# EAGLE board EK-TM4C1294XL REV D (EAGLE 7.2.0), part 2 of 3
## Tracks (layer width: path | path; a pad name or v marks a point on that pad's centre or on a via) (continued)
N$31 (continued)
  Top 0.152: 36.27,24.43 Y1.P$3 36.85,24.42 37.11,24.16 38.1,24.16 38.22,24.19 C44.1 | C44.1 38.48,24.17 | C44.1 38.25,24.16 38.18,24.08 38.18,23.47 38.75,22.9 39.44,22.9 39.55,22.78 43.89,22.78 44.42,23.32 44.45,23.32 U1.P$88
N$32
  Top 0.254: U10.P$15 25.7,41.88 26.29,41.3 26.29,40.01 26.14,39.85 23.24,39.85 22.4,40.69 R32.2
N$33
  Top 0.152: 29.26,29.72 30.25,29.72 31.24,30.71 34.82,30.71 35.51,30.02 37.8,30.02 38.1,29.72 38.4,29.72 U1.P$66 | 29.26,29.72 26.29,29.72 26.16,29.59 Y3.P$1 | 29.26,29.72 29.26,29.38 C48.1
N$34
  Top 0.254: U10.P$10 25.91,48.23 26.98,47.17 26.98,39.7 26.67,39.4 22.25,39.4 22.1,39.55 21.64,39.55 R43.2
N$36
  Top 0.254: R45.1 16.3,40.54 | 16.3,40.54 R46.1 | R43.1 20.66,40.53 | 20.66,40.53 20.65,40.54 | 20.66,40.53 20.69,40.5 | 20.69,40.5 R32.1 | 20.69,40.5 20.65,40.77 19.74,40.77 19.51,40.54 19.13,40.54 | 19.13,40.54 16.3,40.54 | C1.1 19.08,40.49 19.13,40.54
N$44
  Top 0.152: U14.4 7.12,45.2 U14.5
  Top 0.254: U14.4 7.07,45.2 6.1,46.18 5.94,46.18 4.65,44.88 4.65,41.99 5.94,40.69 11.73,40.69 12.45,41.4 R45.2
N$45
  Top 0.152: U14.7 7.12,49.28 U14.8
  Top 0.254: U14.8 7.14,49.28 6.1,48.23 6.02,48.23 3.89,46.1 3.89,42.06 5.94,40.01 15.38,40.01 R46.2
PA0  (via drill 0.3)
  Top 0.152: v64.92,26.09 64.95,26.06 67.74,26.06 69.65,24.16 71.93,24.16 72.06,24.18 JP4.2 | v63.27,43.38 62.94,43.05 56.39,43.05 55.85,43.59 50.06,43.59 49.53,43.05 49,43.05 47.49,41.55 U1.P$33 | v63.5,1.75 62.94,2.29 48.08,2.29 47.55,2.82 43.89,2.82 43.59,3.12 42.75,3.12 42.44,2.82 v32.84,2.82 32.99,2.67
  Bottom 0.152: v63.27,43.38 63.25,43.51 63.25,42.06 64.39,40.92 64.39,34.75 63.63,33.98 63.63,33.68 62.79,32.84 62.79,31.85 62.48,31.55 62.48,27.58 64.01,26.06 64.92,26.06 v64.92,26.09 64.92,21.95 63.86,20.8 63.86,6.71 63.55,6.4 63.55,1.83 63.48,1.75 v63.5,1.75 | v32.84,2.82 32.84,2.36 X11.74
PA1  (via drill 0.3)
  Top 0.152: 45.49,44.27 v45.95,44.27 44.35,44.27 44.12,44.04 42.9,44.04 42.29,44.65 38.94,44.65 37.95,43.66 v37.19,43.66 | v69.27,42.22 58.75,42.22 58.22,42.75 55.85,42.75 55.32,43.28 50.22,43.28 49.68,42.75 49.45,42.75 48.54,41.83 48.54,40.92 48.53,40.92 48.23,40.62 47.85,40.62 47.24,41.22 U1.P$34 46.33,42.14 v46.02,42.14
  Bottom 0.152: v46.02,42.14 46.02,42.6 45.95,42.67 v45.95,44.27 | v37.19,43.66 37.19,43.13 36.88,42.82 36.88,40.23 36.12,39.47 36.12,36.96 35.43,36.27 35.43,33.68 34.98,33.22 33.3,33.22 32.16,32.08 32.16,30.56 31.01,29.41 31.01,27.2 29.03,25.22 29.03,14.86 30.02,13.87 30.02,4.8 30.33,4.5 30.33,2.39 X11.76 | JP5.2 71.88,31.75 69.95,33.68 69.95,41.53 v69.27,42.22
PA2  (via drill 0.3)
  Top 0.152: 44,13.56 R20.2 44.04,13.6 44.04,14.02 44.35,14.33 47.47,14.33 47.62,14.48 v49.61,14.48 50.06,14.48 50.29,14.25 52.2,14.25 53.03,13.41 65.68,13.41 66.29,14.02 68.96,14.02 69.65,13.34 v70.56,13.34 | v117.81,6.78 114.38,6.78 114,6.4 113.23,6.4 113.16,6.33 108.89,6.33 108.58,6.02 106.53,6.02 106.22,5.71 97.16,5.71 96.85,6.02 v96.32,6.02 | v96.01,2.59 v71.02,2.59 | U1.P$35 48.31,39.59 v48.31,39.55
  Bottom 0.152: v48.31,39.55 48.31,39.09 48.16,38.94 48.16,34.59 48.92,33.83 48.92,31.47 49.99,30.4 49.99,29.79 49.23,29.03 49.23,25.45 49.91,24.77 49.91,23.55 49.68,23.32 49.68,14.48 v49.61,14.48 | 118.11,1.29 119.18,2.36 119.18,4.42 118.8,4.8 118.8,5.33 117.81,6.33 v117.81,6.78 | v96.32,6.02 96.32,2.9 v96.01,2.59 | v70.56,13.34 70.56,12.88 70.18,12.5 70.18,4.95 71.02,4.12 v71.02,2.59
  Bottom 0.254: 118.11,1.29 X11.6
PA3  (via drill 0.3)
  Top 0.152: v115.14,5.87 115.06,5.79 113.77,5.79 113.69,5.71 109.35,5.71 109.04,5.41 106.98,5.41 106.68,5.11 94.64,5.11 94.49,5.26 93.57,5.26 93.12,4.8 71.86,4.8 71.4,4.34 70.87,4.34 70.18,5.03 69.49,5.03 69.27,4.8 v68.81,4.8 | v68.73,13.26 68.05,13.26 67.82,13.49 66.6,13.49 66.22,13.11 52.88,13.11 52.05,13.95 50.37,13.95 49.61,13.18 v49.23,13.18 48.84,13.56 48.16,13.56 48.12,13.53 48.19,13.38 R19.2 | v46.94,38.63 46.94,39.17 47.32,39.55 47.32,40.01 U1.P$36
  Bottom 0.152: X11.8 115.57,2.31 114.53,3.35 114.53,4.19 115.14,4.8 v115.14,5.87 | v68.81,4.8 68.73,4.88 v68.73,13.26 | v46.94,38.63 46.94,38.1 47.24,37.8 47.24,33.91 48.01,33.15 48.01,28.19 47.4,27.58 47.4,26.36 48.31,25.45 48.31,22.94 49.07,22.17 49.07,16.38 48.31,15.62 48.31,14.1 v49.23,13.18
PA4  (via drill 0.3)
  Top 0.152: v110.11,47.09 109.65,46.63 107.9,46.63 107.59,46.94 90.3,46.94 88.16,44.81 76.96,44.81 75.59,46.18 70.56,46.18 68.66,44.27 62.71,44.27 62.1,43.66 56.84,43.66 56.31,44.2 49.76,44.2 49.23,43.66 46.94,43.66 46.63,43.36 45.41,43.36 | 45.41,43.36 42.06,43.36 41.76,43.66 41.22,43.66 41.17,43.61 v41.22,43.61 | U1.P$37 46.1,40.69 45.41,41.38 45.41,43.36
  Bottom 0.152: v41.22,43.61 41.22,43.66 40.16,44.73 40.16,51.28 X6.18 | X11.10 113.03,2.16 114.22,3.35 114.22,4.12 113.69,4.65 113.69,6.25 114.07,6.63 114.07,35.81 109.73,40.16 109.73,41.83 109.42,42.14 109.42,46.41 109.5,46.48 v110.11,47.09
PA5  (via drill 0.3)
  Top 0.152: v109.04,47.24 90.14,47.24 88.01,45.11 77.19,45.11 75.82,46.48 70.33,46.48 68.43,44.58 62.41,44.58 61.8,43.97 57.15,43.97 56.62,44.5 49.61,44.5 49.07,43.97 46.63,43.97 46.33,43.66 42.52,43.66 41.99,44.2 40.69,44.2 40.46,43.97 | 40.46,43.97 39.7,43.97 v39.29,43.99 | 40.46,43.97 40.46,43.43 40.92,42.98 44.65,42.98 45.11,42.52 45.11,41.07 45.13,41.07 U1.P$38
  Bottom 0.152: X6.20 36.85,52.05 36.85,51.23 39.32,48.77 39.32,44.5 v39.29,43.99 | X11.12 109.5,2.26 109.5,12.95 110.41,13.87 110.41,22.02 109.35,23.09 109.35,24.23 111.1,25.98 111.1,36.35 109.12,38.33 109.12,46.56 109.04,46.63 v109.04,47.24
PA6  (via drill 0.3)
  Top 0.152: X8.16 104.17,50.83 102.41,50.83 101.65,50.06 98.68,50.06 98.37,50.37 v93.88,50.37 93.57,50.06 90.6,50.06 86.87,46.33 78.11,46.33 76.73,47.7 68.73,47.7 67.13,46.1 58.9,46.1 58.37,45.57 55.78,45.57 55.55,45.8 v44.5,45.8 | v44.12,42.37 43.81,42.06 43.81,40.92 44.12,40.62 44.45,40.62 U1.P$40
  Bottom 0.152: v93.88,50.37 92.73,49.23 92.73,25.91 90.98,24.16 90.98,19.58 94.64,15.93 94.64,14.4 93.04,12.8 93.04,5.71 92.73,5.41 92.73,3.83 X11.25 | v44.12,42.37 44.5,42.75 v44.5,45.8
PA7  (via drill 0.3)
  Top 0.152: v90.14,8.15 89.76,8.53 76.89,8.53 76.58,8.23 72.54,8.23 72.24,8.53 v67.59,8.53 66.98,8.53 66.9,8.46 62.56,8.46 62.03,7.85 54.18,7.85 53.14,8.89 X7.8 | v43.2,41 43.97,40.23 44.27,40.23 U1.P$41 | v43.43,45.49 43.74,45.19 44.96,45.19 45.26,45.49 48.84,45.49 49.15,45.19 58.75,45.19 58.98,45.49 v65.46,45.49
  Bottom 0.152: X11.27 90.14,3.83 v90.14,8.15 | v43.2,41 43.2,42.52 43.51,42.82 43.51,44.5 43.43,44.58 v43.43,45.49 | v65.46,45.49 65.46,36.5 68.66,33.3 68.66,28.19 67.97,27.51 67.97,15.24 67.74,15.01 67.74,12.88 67.89,12.72 67.89,12.34 67.74,12.19 67.74,9.14 67.59,8.99 v67.59,8.53
PB0  (via drill 0.3)
  Top 0.152: v54.79,6.02 54.48,5.79 48.31,5.79 48.23,5.71 42.67,5.71 42.6,5.79 v41.3,5.79 41.22,5.87 | R18.1 18.94,22.63 26.36,22.63 30.79,18.21 36.04,18.21 37.26,19.43 41.76,19.43 v42.06,19.74 43.43,21.11 46.18,21.11 47.19,22.12 U1.P$95
  Bottom 0.152: X11.58 52.07,2.16 53.42,3.5 53.42,4.19 54.79,5.56 v54.79,6.02 | v41.3,5.79 39.93,7.16 39.93,7.92 40.46,8.46 40.46,11.51 41.53,12.57 41.53,13.49 41.15,13.87 41.15,16.08 42.06,16.99 v42.06,19.74
PB2  (via drill 0.3)
  Top 0.152: X8.17 102.62,54.61 101.58,53.57 92.2,53.57 v91.44,52.81 | v91.44,51.51 90.22,51.51 85.95,47.24 78.79,47.24 76.5,49.53 67.97,49.53 66.14,47.7 55.24,47.7 54.79,47.32 v47.55,47.32 v38.56,47.32 | v48.31,26.75 48.31,25.07 47.17,23.93 46.79,23.93 46.25,23.39 46.22,23.39 U1.P$91 | v38.71,5.49 v36.2,5.49
  Bottom 0.152: v91.44,52.81 v91.44,51.51 | v47.55,47.32 47.55,44.2 48.46,43.28 48.46,41.15 47.55,40.23 47.55,39.4 47.85,39.09 47.85,34.37 48.62,33.6 48.62,27.81 48.31,27.51 v48.31,26.75 | X11.67 39.37,4.85 v38.71,5.49 | v36.2,5.49 35.2,6.48 35.2,7.7 35.51,8 35.51,10.82 35.81,11.12 35.81,26.82 36.35,27.36 36.35,27.81 35.36,28.8 35.36,31.17 36.2,32 36.2,36.04 36.73,36.58 36.73,39.09 37.49,39.85 37.49,42.14 38.1,42.75 38.1,44.88 37.87,45.11 37.87,46.63 v38.56,47.32
PB3  (via drill 0.3)
  Top 0.152: X8.19 95.45,54.61 94.79,53.95 91.67,53.95 85.57,47.85 79.32,47.85 77.04,50.14 67.36,50.14 65.53,48.31 54.63,48.31 54.56,48.23 47.09,48.23 46.79,48.54 v46.33,48.54 46.02,48.23 43.97,48.23 43.59,48.62 v38.48,48.62 | v49,24 48.54,24 48.16,23.62 47.01,23.62 U1.P$92
  Bottom 0.152: v46.33,48.54 46.33,44.88 48.08,43.13 48.08,41.38 47.24,40.54 47.24,39.24 47.55,38.94 47.55,34.14 48.31,33.38 48.31,28.04 47.7,27.43 47.7,26.52 48.62,25.6 48.62,25.07 49,24.69 v49,24 | X11.69 36.83,3.86 35.36,5.33 35.05,5.33 34.44,5.94 34.44,7.47 35.13,8.15 35.13,11.2 35.43,11.51 35.43,26.21 34.9,26.75 34.9,31.39 35.81,32.31 35.81,36.2 36.42,36.8 36.42,39.24 37.19,40.01 37.19,42.44 37.8,43.05 37.8,44.65 37.57,44.88 37.57,47.7 v38.48,48.62
PB4  (via drill 0.3)
  Top 0.152: v94.03,12.65 v78.56,12.65 | v94.03,4.65 94.56,4.65 94.72,4.8 106.91,4.8 107.21,5.11 109.19,5.11 109.5,5.41 113.92,5.41 114,5.49 114.68,5.49 114.91,5.26 117.65,5.26 v117.81,5.41 | v78.56,26.75 76.5,26.75 75.29,27.96 71.25,27.96 70.56,27.28 57.84,27.28 57.07,28.04 57.03,28.04 U1.P$121 55.85,29.21 55.85,29.87 56.24,30.25 v56.24,30.94
  Bottom 0.152: v78.56,12.65 78.56,17.6 78.87,17.91 78.87,20.04 78.56,20.34 v78.56,26.75 | v94.03,12.65 v94.03,4.65 | v117.81,5.41 117.81,4.95 118.11,4.65 X11.5 | X6.6 54.61,50.88 53.87,50.14 53.87,44.27 54.41,43.74 54.41,33.07 56.24,31.24 v56.24,30.94
PB5  (via drill 0.3)
  Top 0.152: v116.05,5.87 116.05,6.48 114.83,6.48 114.45,6.1 113.46,6.1 113.39,6.02 109.12,6.02 108.81,5.71 106.76,5.71 106.45,5.41 94.87,5.41 94.72,5.56 93.34,5.56 93.19,5.41 86.87,5.41 86.56,5.11 71.25,5.11 v71.09,5.03 | v69.57,26.67 68.5,26.67 68.2,26.98 57.68,26.98 56.92,27.74 56.77,27.74 U1.P$120 55.47,29.03 55.47,30.1 v54.71,30.86
  Bottom 0.152: X11.7 115.57,5.38 v116.05,5.87 | v71.09,5.03 71.09,8.38 71.48,8.76 71.48,20.88 70.56,21.79 70.56,23.62 71.09,24.16 71.09,25.15 v69.57,26.67 | X6.8 52.07,51.03 52.88,50.22 52.88,43.74 53.49,43.13 53.49,32.16 v54.71,30.86
PC4  (via drill 0.3)  (1 unrouted)
  Top 0.152: v98.22,48.54 100.51,48.54 100.81,48.84 101.88,48.84 102.18,48.54 109.88,48.54 111.18,49.84 v117.96,49.84 | v95.33,37.57 94.87,37.57 94.72,37.72 85.04,37.72 84.2,36.88 78.33,36.88 77.5,37.72 71.09,37.72 67.51,41.3 57.99,41.3 57.91,41.38 52.73,41.38 52.27,40.92 52.27,40.2 U1.P$25
  Bottom 0.152: v98.22,48.54 98.3,40.84 98.3,39.55 96.32,37.57 v95.33,37.57 95.33,31.24 96.62,29.95 96.62,28.42 96.39,28.19 96.39,26.98 96.55,26.82 99.44,23.85 99.44,19.13 95.33,15.01 95.33,3.89 X11.23 | v117.96,49.84 117.96,50.37 119.18,51.59 119.18,53.54 X8.5
PC5  (via drill 0.3)  (1 unrouted)
  Top 0.152: v99.06,47.93 100.43,47.93 101.04,48.54 101.65,48.54 101.96,48.23 110.41,48.23 110.72,48.54 111.33,49.23 v116.74,49.23 | v97.54,37.26 97.08,37.26 96.77,36.96 95.02,36.96 94.56,37.41 85.27,37.41 84.43,36.58 78.11,36.58 77.27,37.41 70.87,37.41 67.28,41 57.76,41 57.68,41.07 52.88,41.07 52.58,40.77 52.58,39.94 U1.P$24
  Bottom 0.152: X8.7 115.57,53.67 116.74,52.5 v116.74,49.23 | v99.06,47.93 99.06,39.01 97.54,37.49 v97.54,37.26 97.54,28.5 100.36,25.68 100.36,18.67 99.9,18.21 99.9,15.54 99.59,15.24 99.59,13.34 98.53,12.27 98.53,5.79 97.54,4.8 97.54,4.04 97.74,3.83 97.77,3.83 X11.21
PC6  (via drill 0.3)  (1 unrouted)
  Top 0.152: v111.48,48.16 111.25,47.93 v101.35,47.93 | v100.81,37.03 100.43,36.65 94.79,36.65 94.34,37.11 85.5,37.11 84.66,36.27 77.8,36.27 76.96,37.11 70.64,37.11 67.06,40.69 57.61,40.69 57.53,40.77 53.11,40.77 52.88,40.54 52.88,39.67 U1.P$23
  Bottom 0.152: X8.9 112.01,53.59 112.01,48.69 v111.48,48.16 | v101.35,47.93 101.35,40.62 101.19,40.46 101.19,37.41 v100.81,37.03 100.81,34.82 100.58,34.52 100.58,27.43 103.1,24.92 103.1,14.33 101.35,12.57 101.35,4.95 100.33,3.94 X11.19
PC7  (via drill 0.3)  (1 unrouted)
  Top 0.152: v101.8,37.49 101.8,36.96 101.19,36.35 94.56,36.35 94.11,36.8 85.72,36.8 84.89,35.97 77.57,35.97 76.73,36.8 70.41,36.8 66.83,40.39 57.45,40.39 57.38,40.46 53.34,40.46 53.19,40.31 53.19,39.41 U1.P$22
  Bottom 0.152: X11.17 102.87,7.09 101.8,8.15 101.8,12.5 103.4,14.1 103.4,25.22 100.97,27.66 100.97,32.38 101.8,33.22 v101.8,37.49 101.5,37.8 101.5,40.08 101.8,40.39 101.8,47.32 101.96,47.47 101.96,49.61 104.09,51.74 104.09,53.29 X8.15
PD0  (via drill 0.3)
  Top 0.152: X9.14 107.95,8.74 107.06,7.85 104.93,7.85 104.62,7.54 99.67,7.54 98.91,8.31 92.73,8.31 91.67,7.24 86.33,7.24 85.72,7.85 84.35,7.85 84.12,7.62 78.41,7.62 77.72,6.93 70.18,6.93 69.49,7.62 66.45,7.62 66.22,7.85 63.86,7.85 v63.25,7.24 | v62.18,32.23 61.87,32.54 58.65,32.54 U1.P$1
  Bottom 0.152: X11.50 63.25,2.36 v63.25,7.24 63.25,8.53 63.55,8.84 63.55,21.03 64.62,22.17 64.62,24.92 62.18,27.36 v62.18,32.23
PD1  (via drill 0.3)
  Top 0.152: X9.12 110.49,8 110.34,7.85 107.67,7.85 107.37,7.54 105.31,7.54 105,7.24 99.52,7.24 98.75,8 92.96,8 91.9,6.93 86.03,6.93 85.42,7.54 84.66,7.54 84.35,7.24 78.56,7.24 77.95,6.63 69.95,6.63 69.34,7.24 v65.84,7.24 | v65.99,33.53 63.78,33.53 63.09,32.84 59.74,32.84 58.9,33.68 58.77,33.68 U1.P$2
  Bottom 0.152: X11.48 64.8,1.29 64.85,1.29 65.84,2.29 v65.84,7.24 65.84,8.46 65.99,8.61 v65.99,33.53
PD2  (via drill 0.3)
  Top 0.152: v60.73,33.45 59.59,33.45 59.05,33.98 58.51,33.98 U1.P$3
  Bottom 0.152: X6.3 58.67,53.09 58.67,51.13 60.5,49.3 v60.73,33.45 60.73,32.46 61.87,31.39 61.87,27.13 64.31,24.69 64.31,22.33 63.25,21.18 61.87,19.81 61.87,4.95 61.19,4.27 61.19,2.77 X11.52
PD3  (via drill 0.3)
  Top 0.152: X8.13 107.95,54.46 106.68,53.19 93.04,53.19 v92.81,52.96 | v92.81,51.44 92.28,50.9 90.22,50.9 86.26,46.94 78.56,46.94 76.5,49 72.39,49 71.7,48.31 68.35,48.31 66.83,46.79 57.76,46.79 57.45,46.48 v56.31,46.48 | 56.16,32.99 v56.27,32.99 56.92,32.99 57.15,33.22 57.18,33.22 U1.P$4 | v57.99,19.89 59.21,19.89 59.66,20.19 v66.75,20.19
  Bottom 0.152: v92.81,52.96 v92.81,51.44 | v66.75,20.19 66.75,13.41 66.52,13.18 66.52,4.65 66.22,4.34 66.22,2.36 X11.46 | v57.99,19.89 57.99,20.5 57.91,20.57 57.91,26.75 56.92,27.74 56.92,31.17 56.24,31.85 56.24,32.92 v56.27,32.99 56.31,33.1 v56.31,46.48
PD4  (via drill 0.3)  (1 unrouted)
  Top 0.152: v73.15,29.18 70.71,29.18 70.03,28.5 60.88,28.5 60.27,29.11 58.22,29.11 U1.P$125
  Bottom 0.152: X11.40 73.84,2.36 73.84,25.58 JP4.3 73.15,28.45 v73.15,29.18
PD5  (via drill 0.3)  (1 unrouted)
  Top 0.152: v74.37,29.18 74.37,29.26 73.84,29.79 70.71,29.79 69.72,28.8 61.11,28.8 60.5,29.41 58.52,29.41 58.37,29.57 58.33,29.57 U1.P$126
  Bottom 0.152: X11.38 76.43,2.31 76.43,5.64 75.59,6.48 75.59,20.19 76.2,20.8 76.2,27.36 v74.37,29.18 73.84,29.72 73.84,33.22 74.91,34.29 JP5.3
PD6  (via drill 0.3)
  Top 0.152: U4.4 77.57,41.45 v77.57,40.54 | v76.96,29.72 74.98,29.72 74.6,30.1 70.03,30.1 v69.34,29.41 69.34,29.49 68.89,29.49 68.5,29.11 61.34,29.11 60.73,29.72 58.75,29.72 58.6,29.87 58.59,29.87 U1.P$127
  Bottom 0.152: v77.57,40.54 77.57,39.85 77.5,39.78 77.5,31.24 76.96,30.71 v76.96,29.72 | v69.34,29.41 69.34,28.35 68.28,27.28 68.28,15.01 68.12,14.86 68.12,13.03 68.43,12.72 68.43,11.73 68.12,11.43 68.12,9.22 68.35,8.99 68.35,8.08 68.12,7.85 68.12,4.5 68.81,3.81 68.81,2.31 X11.44
PD7  (via drill 0.3)
  Top 0.152: X8.14 107.09,52.07 105.54,50.52 102.79,50.52 102.03,49.76 90.91,49.76 87.17,46.02 77.8,46.02 76.43,47.4 68.89,47.4 66.37,44.88 v59.36,44.88 | v60.5,30.86 58.67,30.86 U1.P$128 | X11.42 71.42,1.27 69.95,2.74 58.67,2.74 v58.45,2.97
  Bottom 0.152: v59.36,44.88 59.36,43.81 59.13,43.59 59.13,35.97 59.28,35.81 59.28,32 60.43,30.86 v60.5,30.86 59.82,30.18 59.82,25.38 60.58,24.61 60.58,22.55 61.19,21.95 61.19,7.16 58.45,4.42 v58.45,2.97
PE0  (via drill 0.3)
  Top 0.152: X11.14 109.04,1.27 109.35,1.6 109.96,2.29 117.04,2.29 v117.12,2.21 | v66.06,37.34 65.23,38.18 59.97,38.18 59.21,37.41 55.17,37.41 54.71,36.96 54.69,36.96 U1.P$15 | X8.6 116.18,50.14 110.95,50.14 109.65,48.84 102.49,48.84 102.18,49.15 91.44,49.15 87.71,45.41 77.42,45.41 76.05,46.79 70.1,46.79 68.73,45.41 v68.2,45.41
  Bottom 0.152: X8.6 118.11,51.05 117.27,50.22 117.27,49.61 117.35,49.53 117.35,46.41 116.81,45.87 116.81,44.5 117.04,44.27 117.04,38.25 115.9,37.11 115.9,33.22 118.42,30.71 118.42,25.6 117.65,24.84 117.65,12.57 117.12,12.04 v117.12,2.21 | v66.06,37.34 66.45,37.34 67.28,38.18 67.28,44.5 v68.2,45.41
PE1  (via drill 0.3)
  Top 0.152: X11.16 106.45,1.27 106.91,1.75 107.44,2.29 109.5,2.29 109.8,2.59 116.2,2.59 v116.51,2.9 | v66.67,36.2 66.29,36.2 64.62,37.87 60.12,37.87 59.36,37.11 55.41,37.11 U1.P$14 | X8.8 114.17,50.67 106.83,50.67 105.31,49.15 102.87,49.15 102.56,49.45 91.14,49.45 87.4,45.72 77.65,45.72 76.28,47.09 69.88,47.09 69.49,46.71 v69.04,46.71
  Bottom 0.152: X8.8 116.05,51.59 116.05,48.23 116.43,47.85 116.51,47.78 116.51,44.35 116.74,44.12 116.74,38.48 115.21,36.96 115.21,33.3 118.11,30.4 118.11,25.83 117.35,25.07 117.35,12.8 116.66,12.12 116.66,3.05 v116.51,2.9 | v66.67,36.2 67.67,37.19 67.67,43.43 69.04,44.81 v69.04,46.71
PE2  (via drill 0.3)
  Top 0.152: v103.94,37.72 103.25,37.03 102.49,37.03 101.42,35.97 89.92,35.97 88.7,34.75 76.5,34.75 75.67,35.59 66.29,35.59 64.31,37.57 60.35,37.57 59.59,36.8 55.7,36.8 55.32,36.42 55.24,36.42 55.03,36.2 U1.P$13 | X8.10 112.88,52.07 111.78,50.98 106.53,50.98 105.69,50.14 103.4,50.14 v103.1,49.84
  Bottom 0.152: v103.1,49.84 102.26,49 102.26,42.06 104.24,40.08 104.24,38.02 v103.94,37.72 103.94,2.44 102.87,1.37 X11.18
PE3  (via drill 0.3)
  Top 0.152: v109.8,19.51 109.65,19.36 104.78,19.36 103.56,18.14 v102.18,18.14 | U1.P$12 55.93,36.5 59.74,36.5 60.5,37.26 64.08,37.26 66.06,35.28 75.44,35.28 76.28,34.44 88.92,34.44 90.14,35.66 101.65,35.66 102.64,36.65 103.94,36.65 104.7,37.41 104.7,39.93 106.6,41.83 v108.43,41.83
  Bottom 0.152: X8.12 110.49,50.44 108.36,48.31 108.36,42.75 108.43,42.67 v108.43,41.83 108.43,39.4 108.66,39.17 108.66,38.18 110.8,36.04 110.8,26.36 108.97,24.54 108.97,22.78 109.8,21.95 v109.8,19.51 | v102.18,18.14 101.42,17.37 101.42,14.1 99.21,11.89 99.21,2.39 X11.20
PE4  (via drill 0.3)
  Top 0.152: v100.81,17.53 115.21,17.53 116.59,16.15 v119.33,16.15 | 79.4,27.43 v79.32,27.43 76.43,27.43 75.59,28.27 70.94,28.27 70.56,27.89 60.5,27.89 59.89,28.5 57.7,28.5 U1.P$123 | v101.35,24.61 100.13,25.83 98.98,25.83 98.68,26.14 92.51,26.14 89.46,23.09 v79.4,23.09
  Bottom 0.152: X8.3 120.52,54.61 119.56,53.65 119.56,51.44 118.57,50.44 118.57,45.95 118.34,45.72 118.34,38.79 120.17,36.96 120.17,31.62 118.72,30.18 118.72,16.76 v119.33,16.15 | X11.22 98.83,2.31 98.83,12.04 100.81,14.02 v100.81,17.53 101.35,18.06 101.35,18.21 102.49,19.36 102.49,23.47 v101.35,24.61 | v79.4,23.09 79.4,27.36 v79.32,27.43
PE5  (via drill 0.3)
  Top 0.152: v108.05,29.34 108.05,28.88 105.99,26.82 101.8,26.82 100.66,27.96 99.14,27.96 98.6,27.43 v97.08,27.43 91.21,27.43 90.68,27.96 79.7,27.96 79.63,28.04 79.02,28.04 78.94,27.96 76.43,27.96 75.82,28.57 70.64,28.57 70.26,28.19 60.66,28.19 60.05,28.8 57.99,28.8 57.76,29.03 57.73,29.03 U1.P$124
  Bottom 0.152: X8.11 109.5,53.62 109.5,50.06 108.05,48.62 108.05,42.6 107.52,42.06 107.52,41.6 108.05,41.07 108.05,38.79 108.36,38.48 108.36,35.74 109.65,34.44 109.65,30.86 108.13,29.34 v108.05,29.34 | v97.08,27.43 97.08,26.9 99.75,24.23 99.75,18.97 99.29,18.52 99.29,18.36 97.23,16.31 97.23,4.72 96.77,4.19 96.77,1.83 96.24,1.29 95.63,1.29 95.56,1.22 X11.24
PF0  (via drill 0.3)
  Top 0.152: D4.A 32.91,6.24 v33.3,6.63 33.38,6.71 39.4,6.71 v40.39,5.71 | v39.09,13.79 34.82,13.79 34.67,13.79 v33.3,13.79 | v41.38,41.91 41.99,41.3 41.99,41 42.22,40.77 43.05,39.85 44.09,39.85 U1.P$42
  Bottom 0.152: v39.09,13.79 39.09,14.63 38.86,14.86 38.86,18.9 40.01,20.12 40.92,21.03 40.92,22.86 40.01,23.77 40.01,33.68 41.07,34.75 41.07,36.73 40.54,37.26 40.54,40.23 41.38,41.07 v41.38,41.91 | v33.3,13.79 33.3,10.29 33.38,10.21 33.38,7.32 33.3,7.24 v33.3,6.63 | X11.66 41.91,1.91 40.62,3.2 40.62,5.49 v40.39,5.71
PF1  (via drill 0.3)
  Top 0.152: X9.1 123.19,13.44 121.08,15.54 116.51,15.54 114.83,17.22 101.88,17.22 101.58,16.92 98.6,16.92 97.99,16.31 93.12,16.31 92.89,16.08 v92.05,16.08 | v90.53,31.55 89.92,31.55 89.53,31.17 81.46,31.17 81,30.71 69.04,30.71 68.12,29.79 63.48,29.79 61.49,31.77 56.69,31.77 56.39,32.08 54.86,32.08 54.33,32.61 52.43,32.61 52.12,32.92 46.79,32.92 v46.25,32.38 | v46.18,38.18 45.72,38.18 45.57,38.02 45.34,38.02 45.26,38.1 45.26,38.11 U1.P$43 | v47.85,18.97 47.55,18.67 44.04,18.67 43.28,17.91 38.86,17.91 v38.25,17.3
  Bottom 0.152: v92.05,16.08 90.37,17.75 90.37,24.46 91.29,25.38 91.29,26.67 91.06,26.9 91.06,30.18 90.53,30.71 v90.53,31.55 | v46.18,38.18 46.18,37.64 45.95,37.41 45.95,36.73 46.63,36.04 46.63,32.77 v46.25,32.38 46.79,31.85 46.79,31.39 46.33,30.94 46.33,26.06 47.4,24.99 47.4,22.4 48.16,21.64 48.16,19.81 47.85,19.51 v47.85,18.97 | v38.25,17.3 38.25,12.88 38.33,12.8 38.33,6.86 38.1,6.63 38.1,5.03 38.33,4.8 38.33,3.35 38.63,3.05 38.63,1.98 39.34,1.27 X11.68
PF2  (via drill 0.3)
  Top 0.152: 120.62,11.4 120.62,12.27 119.41,13.49 117.88,13.49 114.45,16.92 102.11,16.92 101.5,16.31 v98.98,16.31 | v96.77,30.79 88.09,30.79 88.01,30.86 81.69,30.86 81.23,30.4 69.27,30.4 68.35,29.49 63.25,29.49 61.27,31.47 56.54,31.47 56.24,31.77 54.56,31.77 54.03,32.31 52.2,32.31 51.89,32.61 47.7,32.61 v47.4,32.31 | v46.56,37.11 46.1,37.57 45.24,37.57 U1.P$44 | v44.58,6.33 43.28,6.33 43.2,6.4 40.31,6.4 39.4,7.32 v37.72,7.32 | 120.62,11.35 120.62,11.4 | 120.62,11.4 X9.3
  Bottom 0.152: v98.98,16.31 98.98,17.37 99.59,17.98 99.59,18.36 100.05,18.82 100.05,25.45 96.93,28.57 96.93,30.63 v96.77,30.79 | v46.56,37.11 46.94,36.73 46.94,32.77 v47.4,32.31 47.4,31.47 46.63,30.71 46.63,26.21 47.7,25.15 47.7,22.63 48.46,21.87 48.46,16.69 46.02,14.25 46.02,11.96 45.87,11.81 45.87,10.97 46.33,10.52 46.33,9.68 45.87,9.22 45.87,7.62 v44.58,6.33 | v37.72,7.32 37.72,4.65 38.02,4.34 38.02,1.68 37.8,1.45 37.34,1.45 37.29,1.4 37.11,1.4 X11.70
PF3  (via drill 0.3)
  Top 0.152: X9.5 113.84,15.7 v93.88,15.7 | v90.22,45.87 89.76,45.34 89.23,45.34 88.39,44.5 76.81,44.5 75.44,45.87 70.79,45.87 68.89,43.97 62.94,43.97 62.33,43.36 56.54,43.36 56.01,43.89 49.91,43.89 49.38,43.36 47.62,43.36 v47.09,42.82 | v45.19,36.96 45.19,37.03 44.1,38.12 U1.P$45 | v34.75,32.23 36.42,32.23 37.11,31.55 39.47,31.55 39.55,31.47 44.42,31.47 44.73,31.77 45.34,31.77 45.41,31.85 v45.49,31.85
  Bottom 0.152: v90.22,45.87 90.22,39.09 92.2,37.11 92.2,31.39 91.36,30.56 91.36,27.81 91.59,27.58 91.59,25.22 90.68,24.31 90.68,18.9 v93.88,15.7 | v47.09,42.82 46.71,42.44 46.71,40.69 45.19,39.17 v45.19,36.96 46.25,35.89 46.25,33.3 45.49,32.54 v45.49,31.85 45.41,31.85 | X11.72 34.29,2.29 35.28,3.28 35.28,4.57 34.06,5.79 34.06,19.43 34.52,19.89 34.52,31.55 34.75,31.77 v34.75,32.23
PF4  (via drill 0.3)
  Top 0.152: X11.64 44.45,1.4 44.27,1.37 44.2,1.45 43.28,1.45 42.44,2.29 38.79,2.29 38.56,2.06 37.64,2.06 37.41,2.29 33.38,2.29 33.22,2.13 32.54,2.13 32.38,2.29 28.35,2.29 v27.96,1.91 | v27.96,6.1 29.07,6.1 D3.A | v45.03,36.04 45.03,36.2 44.58,36.65 44.58,37.11 U1.P$46 | v44.73,32.38 44.2,32.38 44.04,32.23 43.36,32.23 42.9,31.77 39.78,31.77 39.7,31.85 37.41,31.85 36.35,32.92 34.59,32.92 34.14,32.46 34.14,32.31 33.76,31.93 31.85,31.93 v30.86,32.92
  Bottom 0.152: v27.96,1.91 v27.96,6.1 27.96,6.63 27.81,6.78 27.81,12.65 27.05,13.41 27.05,26.36 28.04,27.36 29.57,28.88 29.57,29.79 30.86,31.09 v30.86,32.92 | v45.03,36.04 45.87,35.2 45.87,33.45 44.81,32.38 v44.73,32.38
PG0  (via drill 0.3)
  Top 0.152: 115.59,11.43 111.63,15.39 98.15,15.39 97.84,15.09 93.34,15.09 92.96,15.47 90.3,15.47 87.86,17.91 86.64,17.91 v86.33,18.21 86.18,18.21 85.88,17.91 80.54,17.91 79.78,18.67 79.02,18.67 77.95,17.6 76.5,17.6 76.2,17.91 73.69,17.91 73.3,18.29 70.18,18.29 69.88,18.59 69.04,18.59 68.81,18.36 52.5,18.36 51.89,18.97 49.23,18.97 48.31,19.89 46.86,19.89 v46.63,19.58 | 43.81,36.16 v44.12,36.04 | v44.12,36.04 43.97,36.04 44.08,36.09 v44.12,36.04 | U1.P$49 43.94,36.04 v44.12,36.04
  Top 0.254: 115.59,11.43 X9.7
  Bottom 0.152: v86.33,18.21 86.33,17.53 86.11,17.3 86.11,13.49 85.42,12.8 85.42,7.47 85.65,7.24 85.65,6.55 85.11,6.02 85.11,3.83 X11.31 | v46.63,19.58 46.63,22.55 45.72,23.47 45.72,25.76 45.64,25.83 45.64,28.04 45.11,28.57 45.11,31.17 44.12,32.16 44.12,32.69 44.58,33.15 45.03,33.15 45.41,33.53 45.41,35.2 45.26,35.36 44.81,35.36 v44.12,36.04
PG1  (via drill 0.3)
  Top 0.152: v87.63,12.04 87.55,11.96 62.87,11.96 62.71,12.12 60.38,12.12 X7.1 | v57,32.38 55.09,32.38 53.65,33.83 51.82,33.83 50.29,35.43 43.66,35.43 43.28,35.81 43.28,36.12 42.69,36.71 U1.P$50 | v59.82,16.54 59.51,16.84 58.06,16.84 v57.76,16.54
  Bottom 0.152: X11.29 v87.63,12.04 | v57,32.38 57,31.62 57.23,31.39 57.23,27.89 58.22,26.9 58.22,20.95 58.6,20.57 58.6,18.36 57.76,17.53 57.76,16.56 57.73,16.56 v57.76,16.54 | X7.1 60.27,12.01 60.27,16.08 v59.82,16.54
PH0  (via drill 0.3)
  Top 0.152: v113.16,7.01 112.78,6.63 108.66,6.63 108.36,6.33 106.3,6.33 105.99,6.02 98.91,6.02 98.15,6.78 94.03,6.78 92.96,5.71 82.07,5.71 81.15,6.63 78.87,6.63 78.26,6.02 63.02,6.02 62.1,6.93 54.1,6.93 53.57,6.4 49.23,6.4 48.39,7.24 46.02,7.24 45.72,7.54 43.66,7.54 43.59,7.62 v43.13,7.62 | 50.44,40.69 50.44,40.62 | v49.15,38.33 49.15,39.55 49.53,39.93 49.76,39.93 50.44,40.61 50.44,40.62 | v48.84,34.82 48.54,35.13 45.72,35.13 45.34,34.75 v44.81,34.75 | U1.P$29 50.44,40.62
  Bottom 0.152: 112.93,3.81 X11.9 | 113.08,3.81 113.16,3.89 v113.16,7.01 | v43.13,7.62 43.43,7.92 43.43,10.41 X7.13 44.42,11.58 44.42,11.43 43.66,12.19 43.66,15.09 45.03,16.46 45.03,22.02 44.42,22.63 44.42,24.84 43.66,25.6 43.66,27.81 44.5,28.65 44.5,30.86 43.51,31.85 43.51,32.99 44.2,33.68 44.2,34.21 44.73,34.75 v44.81,34.75 | v49.15,38.33 49.15,37.87 48.46,37.19 48.46,35.2 v48.84,34.82 48.92,34.82
  Bottom 0.254: 113.08,3.81 X11.9
PH1  (via drill 0.3)
  Top 0.152: v112.24,7.24 111.94,6.93 108.43,6.93 108.13,6.63 106.07,6.63 105.77,6.33 99.06,6.33 98.3,7.09 93.8,7.09 92.73,6.02 82.3,6.02 81.38,6.93 78.72,6.93 78.11,6.33 63.25,6.33 62.33,7.24 53.87,7.24 53.34,6.71 49.38,6.71 48.54,7.54 46.25,7.54 45.95,7.85 43.97,7.85 43.51,8.31 42.9,8.31 42.37,7.77 v40.92,7.77 | v42.44,45.57 43.13,44.88 45.11,44.88 45.41,45.19 46.48,45.19 46.79,44.88 v48.31,44.88 | v48.92,40.39 49.63,40.39 U1.P$30
  Bottom 0.152: X11.11 110.57,3.81 110.49,4.42 X11.11 | X11.11 111.48,4.8 111.48,6.48 v112.24,7.24 | v40.92,7.77 40.92,10.44 X7.15 42.67,12.19 42.98,12.19 42.98,15.47 43.89,16.38 43.89,19.96 43.81,20.04 43.81,20.65 44.12,20.95 44.12,24.54 43.36,25.3 43.36,27.96 44.2,28.8 44.2,30.71 43.2,31.7 43.2,33.15 43.89,33.83 43.89,35.36 43.43,35.81 43.43,36.58 44.58,37.72 44.58,38.79 42.6,40.77 42.6,42.44 43.2,43.05 43.2,44.2 42.44,45.03 v42.44,45.57 | v48.31,44.88 48.31,44.35 48.84,43.81 48.84,40.39 v48.92,40.39
PH2  (via drill 0.3)
  Top 0.152: v118.64,6.4 118.64,5.11 118.34,4.8 115.14,4.8 114.61,4.27 114.07,4.27 113.54,4.8 109.96,4.8 109.04,3.89 108.03,3.89 X11.13 | v102.41,16.31 114.38,16.31 117.81,12.88 v119.02,12.88 | v98.98,37.57 98.37,38.18 94.94,38.18 94.79,38.02 84.81,38.02 83.97,37.19 78.56,37.19 77.72,38.02 71.32,38.02 67.74,41.6 58.14,41.6 57.61,42.14 55.24,42.14 54.71,42.67 50.67,42.67 50.52,42.52 50.52,41.83 U1.P$31
  Bottom 0.152: v118.64,6.4 118.64,8.36 X9.6 119.18,9.96 119.18,12.12 119.02,12.27 v119.02,12.88 | 98.98,37.49 v98.98,37.57 98.98,36.73 98.68,36.42 98.68,33.76 100.28,32.16 100.28,27.13 102.79,24.61 102.79,17.75 102.41,17.37 v102.41,16.31
PH3  (via drill 0.3)
  Top 0.152: 105.41,3.83 X11.15 106.45,3.81 107.44,4.8 109.5,4.8 109.8,5.11 114.15,5.11 v114.38,4.88 | U1.P$32 49.45,41.73 49.45,41.99 50.44,42.98 55.02,42.98 55.55,42.44 57.91,42.44 58.45,41.91 67.97,41.91 71.55,38.33 77.95,38.33 78.79,37.49 83.74,37.49 84.58,38.33 94.49,38.33 94.64,38.48 98.22,38.48 102.18,42.44 v110.03,42.44
  Bottom 0.152: X9.8 114.99,8.31 114.99,6.63 114.38,6.02 v114.38,4.88 | 115.59,8.91 X9.8 | X11.15 105.39,3.81 105.31,3.89 | X9.8 114.53,9.93 114.53,35.81 110.03,40.31 v110.03,42.44
PJ0  (via drill 0.3)
  Top 0.152: USR_SW1.P$2 6.33,7.62 6.55,7.39 v7.62,7.39 8.91,6.1 15.32,6.1 v19.36,10.13 19.81,10.13 20.88,11.2 23.39,11.2 27.96,15.77 41.07,15.77 41.68,16.38 44.42,16.38 45.19,17.14 50.67,17.14 51.36,16.46 54.41,16.46 v54.71,16.15 | v52.65,30.4 52.73,29.26 53.72,28.27 53.95,28.27 55.01,27.21 U1.P$116 | USR_SW1.P$1 6.38,15.32 6.71,15.32 6.71,15.47 v8.38,15.47
  Bottom 0.152: X11.82 20.57,2.29 20.57,5.56 19.36,6.78 v19.36,10.13 | v52.65,30.4 52.73,30.33 52.73,29.72 54.06,28.38 54.06,24.73 54.03,24.69 54.03,23.32 55.02,22.33 55.02,16.99 54.71,16.69 v54.71,16.15 | v8.38,15.47 8.38,14.25 7.62,13.49 v7.62,7.39
PJ1  (via drill 0.3)  (1 unrouted)
  Top 0.152: v55.93,16.46 55.55,16.76 51.51,16.76 50.83,17.45 44.96,17.45 44.2,16.69 41.45,16.69 40.84,16.08 27.74,16.08 23.16,11.51 19.2,11.51 18.52,10.82 v14.25,10.82 14.25,8.59 USR_SW2.P$2 | v14.25,12.65 14.25,13.95 14.55,14.51 USR_SW2.P$1 | v54.03,30.25 54.03,29.79 54.1,29.72 54.1,28.7 U1.P$117
  Bottom 0.152: X11.84 17.98,2.34 v17.98,10.82 | v14.25,10.82 v14.25,12.65 | v55.93,16.46 56.24,16.76 56.24,18.75 55.63,19.36 55.63,22.63 57,24 57,25.53 55.55,26.9 55.55,29.03 55.47,29.11 54.63,29.11 54.25,29.49 54.25,30.18 54.18,30.25 v54.03,30.25
PK0  (via drill 0.3)
  Top 0.152: v68.28,36.27 68.28,36.35 68.12,36.5 68.12,36.58 65.53,39.17 56.84,39.17 56.77,39.24 54.56,39.24 54.41,39.09 54.41,38.37 U1.P$18 53.58,37.57 52.27,36.27 v52.27,35.97 | v70.79,10.52 v92.05,10.52
  Bottom 0.152: X11.26 91.67,2.31 91.67,10.13 v92.05,10.52 | v52.27,35.97 52.27,36.42 53.19,37.34 53.19,42.9 52.58,43.51 52.5,49.99 50.49,51.99 49.61,51.99 X6.10 | 68.58,35.97 v68.28,36.27 69.27,35.28 69.27,32.92 70.03,32.16 70.03,28.57 68.58,27.13 68.58,23.24 69.72,23.24 70.26,22.71 70.26,21.57 71.17,20.65 71.17,11.43 70.79,11.05 v70.79,10.52
PK1  (via drill 0.3)
  Top 0.152: v88.92,36.12 87.86,35.05 76.81,35.05 75.97,35.89 69.88,35.89 66.29,39.47 57,39.47 56.92,39.55 54.18,39.55 54.1,39.47 54.1,38.63 U1.P$19 52.12,36.65 | 52.12,36.65 | 52.12,36.65 51.97,36.5 51.74,36.5 v51.28,36.04 51.13,35.89
  Bottom 0.152: X11.28 91.29,2.39 91.29,14.55 89.76,16.08 89.76,33.15 88.92,33.98 v88.92,36.12 | X6.12 48.01,51.05 50.9,51.05 52.2,49.76 52.2,43.43 52.88,42.75 52.88,37.64 v51.28,36.04
PK2  (via drill 0.3)
  Top 0.152: v87.71,36.12 87.02,36.12 86.26,35.36 77.04,35.36 76.2,36.2 70.03,36.2 66.45,39.78 57.15,39.78 57.07,39.85 53.95,39.85 53.8,39.7 53.8,38.89 U1.P$20 51.86,36.96 v51.28,36.96
  Bottom 0.152: 87.71,36.27 v87.71,36.12 87.71,34.59 89.46,32.84 89.46,15.85 90.53,14.78 90.53,11.43 89.15,10.06 89.15,2.79 X11.30 | v51.28,36.96 52.58,38.25 52.58,42.6 51.89,43.28 51.89,49.61 50.75,50.75 45.77,50.75 X6.14
PK3  (via drill 0.3)
  Top 0.152: 86.11,36.12 v86.03,36.12 85.57,36.12 85.11,35.66 77.34,35.66 76.5,36.5 70.18,36.5 66.6,40.08 57.3,40.08 57.23,40.16 53.65,40.16 53.49,40.01 53.49,39.15 U1.P$21 51.98,37.64 51.74,37.64 51.66,37.64 v51.36,37.95 | v50.29,50.14 49.68,50.75 43.2,50.75 41.91,52.05 X6.16
  Bottom 0.152: v86.03,36.12 86.03,35.66 89.15,32.54 89.15,20.04 89,19.89 89,15.85 90.14,14.71 90.14,11.58 88.85,10.29 88.85,3.35 87.78,2.29 86.11,2.29 X11.32 | v50.29,50.14 51.59,48.84 51.59,43.13 52.27,42.44 52.27,39.32 51.36,38.41 51.36,38.1 51.51,37.95 | 51.51,37.95 51.59,37.95 | 51.51,37.95 v51.36,37.95
PK4  (via drill 0.3)
  Top 0.152: v26.67,34.06 26.67,34.52 28.12,35.97 30.4,35.97 31.93,34.44 32.23,34.44 32.77,33.91 v34.52,33.91 35.28,33.91 35.66,33.53 37.19,33.53 37.41,33.76 38.3,33.76 U1.P$63 | v57.53,44.58 57.07,44.58 56.84,44.81 49.38,44.81 48.84,44.27 46.86,44.27 46.25,44.88 45.64,44.88 45.34,44.58 42.98,44.58 42.6,44.96 38.25,44.96 37.95,44.65 v36.96,44.65
  Bottom 0.152: 57.15,11.35 X7.3 58.37,12.65 58.37,17.45 58.9,17.98 58.9,20.8 58.52,21.18 58.52,27.13 58.75,27.36 58.75,28.27 58.52,28.5 58.52,32.31 57.53,33.3 57.53,36.88 58.37,37.72 58.37,41.45 57.53,42.29 v57.53,44.58 | v26.67,34.06 26.67,12.95 26.52,12.8 26.52,11.89 26.67,11.73 X11.77 | v36.96,44.65 36.58,44.27 36.58,40.39 34.82,38.63 34.82,34.21 v34.52,33.91
PK5  (via drill 0.3)
  Top 0.152: v55.24,14.33 53.03,14.33 52.43,14.94 50.52,14.94 49.84,15.62 47.4,15.62 46.71,14.94 43.05,14.94 41.53,13.41 40.46,13.41 40.23,13.18 37.57,13.18 37.34,13.41 35.89,13.41 35.59,13.11 v29.41,13.11 | v52.81,33.22 43.66,33.22 42.52,32.08 39.93,32.08 39.85,32.16 39.85,32.77 U1.P$62
  Bottom 0.152: X7.5 54.61,13.89 v55.24,14.33 55.24,15.32 55.32,15.39 55.32,22.78 56.69,24.16 56.69,25.3 55.17,26.75 55.17,27.96 53.42,29.72 53.42,31.62 52.96,32.08 52.96,32.61 52.81,32.77 v52.81,33.22 | v29.41,13.11 29.41,4.01 X11.75
PK6  (via drill 0.3)
  Top 0.152: X7.17 40.39,11.43 41.38,10.44 45.34,10.44 v45.72,10.06 | v40.69,32.69 40.16,32.69 40.16,32.99 39.58,33.58 U1.P$61
  Bottom 0.152: v45.72,10.06 45.72,9.53 45.49,9.3 45.49,8.31 43.66,6.48 43.66,4.65 44.42,3.89 44.45,4.14 | 44.5,4.19 44.45,4.14 | 44.45,4.14 X11.63 | v40.69,32.69 40.69,31.93 41.38,31.24 41.38,30.48 40.31,29.41 40.31,23.93 41.22,23.01 41.22,20.8 39.17,18.75 39.17,15.09 39.93,14.33 39.93,11.99 X7.17
PK7  (via drill 0.3)
  Top 0.152: v35.81,7.32 36.27,7.77 37.26,7.77 37.41,7.92 38.1,7.92 38.18,7.85 39.32,7.85 40.46,6.71 43.59,6.71 43.81,6.93 45.26,6.93 45.57,6.63 47.24,6.63 v47.55,6.33 | v41.6,32.77 41.07,33.3 40.46,33.3 U1.P$60 | v40.77,12.8 40.46,12.5 37.87,12.5 37.87,12.47 X7.19
  Bottom 0.152: X7.19 36.8,11.43 35.81,10.44 v35.81,7.32 | X11.59 49.53,5.56 48.77,6.33 v47.55,6.33 | v41.6,32.77 41.6,31.55 41.68,31.47 41.68,30.33 40.62,29.26 40.62,24.08 41.53,23.16 41.53,20.57 39.47,18.52 39.47,16.69 40.77,15.39 v40.77,12.8
PL0  (via drill 0.3)
  Top 0.152: X9.13 107.9,11.48 107.9,11.89 105.92,13.87 105.08,13.87 104.78,13.56 96.16,13.56 95.86,13.87 93.27,13.87 92.96,13.56 89.15,13.56 88.7,14.02 88.7,14.48 87.78,15.39 80.7,15.39 79.86,14.55 v69.88,14.55 65.84,14.55 65,13.72 54.79,13.72 54.71,13.79 53.11,13.79 52.27,14.63 50.37,14.63 49.68,15.32 47.55,15.32 46.86,14.63 43.43,14.63 43.2,14.4 43.2,13.34 42.67,12.8 v42.22,12.8 | v42.75,24.61 42.75,25.07 42.67,25.15 42.67,25.53 43.23,26.08 U1.P$81
  Bottom 0.152: v69.88,14.55 69.88,3.83 X11.43 | v42.75,24.61 42.75,20.19 42.67,20.12 42.67,17.07 41.45,15.85 41.45,14.86 41.83,14.48 41.83,13.18 v42.22,12.8
PL1  (via drill 0.3)
  Top 0.152: X9.15 104.27,12.57 95.17,12.57 94.49,13.26 93.73,13.26 93.42,12.95 79.17,12.95 78.87,13.26 78.18,13.26 77.19,12.27 67.97,12.27 67.67,12.57 v67.21,12.57 66.75,12.57 66.45,12.27 63.09,12.27 62.87,12.5 51.51,12.5 v50.67,13.34 | v49.91,28.8 48.01,28.8 47.85,28.65 44.88,28.65 44.12,27.89 44.12,26.39 U1.P$82
  Bottom 0.152: v67.21,12.57 67.21,9.53 66.9,9.22 66.9,7.77 67.28,7.39 67.28,3.83 X11.45 | v50.67,13.34 50.67,15.24 49.99,15.93 49.99,23.16 50.22,23.39 50.22,24.99 49.53,25.68 49.53,28.42 v49.91,28.8
PL2  (via drill 0.3)
  Top 0.152: X9.17 102.03,11.43 100.89,10.29 99.75,10.29 98.91,11.12 65.53,11.12 65.38,10.97 v64.77,10.97 | v44.96,27.81 44.42,27.28 44.42,26.12 U1.P$83 | v45.49,15.54 45.8,15.24 46.56,15.24 47.24,15.93 49.99,15.93 50.67,15.24 52.58,15.24 53.19,14.63 54.56,14.63 54.86,14.94 57.99,14.94 58.52,14.33 63.09,14.33 63.86,14.94 v64.77,14.94
  Bottom 0.152: X11.47 v64.77,10.97 v64.77,14.94 | v44.96,27.81 44.42,27.28 44.42,26.14 44.58,25.98 44.58,25.76 45.03,25.3 45.03,23.16 45.72,22.4 45.72,16.23 45.49,16 v45.49,15.54
PL3  (via drill 0.3)
  Top 0.152: X9.19 65.53,11.43 65.3,11.66 64.31,11.66 64.08,11.43 v62.48,11.43 62.41,11.35 | v46.33,15.93 46.63,16.23 50.14,16.23 50.83,15.54 52.73,15.54 53.34,14.94 54.33,14.94 54.63,15.24 58.22,15.24 58.75,14.63 59.66,14.63 59.97,14.94 v62.64,14.94 | U1.P$84 45.03,26.17 v45.03,26.67
  Bottom 0.152: X11.49 62.26,10.44 62.48,10.67 62.48,11.2 62.23,11.46 62.23,11.3 v62.48,11.43 | v45.03,26.67 45.03,25.83 45.34,25.53 45.34,23.39 46.02,22.63 46.02,16.69 46.33,16.38 v46.33,15.93 | v62.64,14.94 62.64,13.87 62.48,13.64 v62.48,11.43 | 62.64,11.58 v62.48,11.43
PL4  (via drill 0.3)
  Top 0.152: X9.9 109.98,14.48 104.62,14.48 104.32,14.17 96.7,14.17 96.39,14.48 v92.28,14.48 | v90.37,26.14 88.85,26.14 88.24,25.53 82.3,25.53 82.22,25.45 80.01,25.45 75.67,21.11 68.43,21.11 68.12,21.41 58.22,21.41 57.45,22.17 54.03,22.17 53.72,21.87 v53.03,21.87 | v51.44,28.19 47.62,28.19 47.4,27.96 44.96,25.53 U1.P$85 | X11.65 42.9,4.8 50.52,4.8 v50.83,4.5
  Bottom 0.152: v92.28,14.48 91.82,14.48 90.07,16.23 90.07,25.3 90.37,25.6 v90.37,26.14 90.37,26.29 | 53.03,21.79 52.05,22.78 52.05,25.68 51.36,26.36 v51.44,28.19 | v50.83,4.5 49.99,5.33 49.99,7.77 50.52,8.31 50.52,9.45 50.83,9.75 50.83,11.81 51.51,12.5 52.05,12.5 52.5,12.95 52.5,16.54 53.72,17.75 53.72,20.57 53.03,21.26 53.03,21.79 | 53.03,21.79 v53.03,21.87
PL5  (via drill 0.3)
  Top 0.152: X9.11 107.75,14.17 104.85,14.17 104.55,13.87 96.47,13.87 96.16,14.17 92.89,14.17 92.58,13.87 91.82,13.87 91.52,14.17 v89.53,14.17 | v88.47,20.34 79.17,20.34 78.49,21.03 77.04,21.03 75.89,19.89 68.2,19.89 67.59,19.28 53.57,19.28 v53.11,19.74 | v50.75,27.51 50.06,27.51 49.68,27.89 47.78,27.89 45.34,25.45 45.34,25.38 44.67,24.7 U1.P$86 43.92,23.93 v43.43,23.93 | v42.06,15.32 41.76,15.01 28.73,15.01 26.14,12.42 26.14,11.81 25.91,11.58 v24.69,11.58
  Bottom 0.152: v89.53,14.17 89.53,14.78 88.7,15.62 88.7,19.66 88.47,19.89 v88.47,20.34 | v53.11,19.74 52.12,19.74 51.36,20.5 51.36,22.25 51.59,22.48 51.59,25.6 50.75,26.44 v50.75,27.51 | v43.43,23.93 43.43,23.32 43.2,23.09 43.2,16.23 42.29,15.32 v42.06,15.32 | v24.69,11.58 24.69,8 24.23,7.54 24.23,3.91 X11.79
PM0  (via drill 0.3)
  Top 0.152: X7.7 52.12,11.43 53.11,10.44 63.93,10.44 64.08,10.29 65.3,10.29 65.46,10.44 69.57,10.44 70.26,9.75 72.24,9.75 72.39,9.6 v72.39,9.68 | v52.05,31.62 51.59,31.17 51.59,30.25 50.83,29.49 48.16,29.49 47.62,28.96 44.73,28.96 43.43,27.66 43.13,27.66 U1.P$78
  Bottom 0.152: v72.39,9.68 X11.41 | v52.05,31.62 51.74,31.32 51.74,29.72 53.34,28.12 53.34,26.06 52.35,25.07 52.35,23.39 53.72,22.02 53.72,21.03 54.03,20.73 54.03,17.53 52.81,16.31 52.81,12.8 52.07,12.06 X7.7
PM1  (via drill 0.3)
  Top 0.152: v74.98,8.84 74.68,8.53 72.77,8.53 72.47,8.84 70.56,8.84 69.27,10.13 65.68,10.13 65.53,9.98 63.93,9.98 63.78,10.13 50.9,10.13 49.61,11.43 X7.9 49.53,11.35 | v49.38,30.1 48.08,30.1 47.24,29.26 44.58,29.26 43.36,28.04 42.95,28.04 U1.P$77
  Bottom 0.152: v74.98,8.84 74.98,3.86 X11.39 | v49.38,30.1 48.92,29.64 48.92,25.22 49.61,24.54 49.61,23.7 49.38,23.47 49.38,16.23 49,15.85 49,14.17 49.3,13.87 49.45,13.87 49.91,13.41 49.91,12.8 49.53,12.42 X7.9
PM2  (via drill 0.3)
  Top 0.152: X7.11 47.14,11.23 47.14,10.62 48.23,9.53 48.69,9.53 49.07,9.91 50.6,9.91 51.05,9.45 51.05,8.38 51.59,7.85 52.5,7.85 52.96,8.31 53.26,8.31 54.03,7.54 62.33,7.54 62.87,8.15 66.45,8.15 66.67,7.92 69.72,7.92 70.41,7.24 76.66,7.24 76.96,7.54 v77.42,7.54 | v47.32,30.56 47.24,30.56 46.79,30.1 44.96,30.1 43.2,28.35 42.69,28.35 U1.P$76
  Bottom 0.152: X11.37 77.47,7.49 v77.42,7.54 | v47.32,30.56 47.02,30.25 47.02,26.29 48.01,25.3 48.01,22.78 48.77,22.02 48.77,16.54 46.33,14.1 46.33,12.12 46.99,11.46 X7.11
PM3  (via drill 0.3)
  Top 0.152: v82.6,6.63 84.35,6.63 84.66,6.33 92.43,6.33 93.5,7.39 98.45,7.39 99.21,6.63 105.54,6.63 105.84,6.93 107.9,6.93 108.2,7.24 111.33,7.24 111.94,7.85 118.57,7.85 119.61,8.89 X9.4 | v80.01,16.61 75.89,16.61 75.21,17.22 73.3,17.22 72.85,17.68 70.18,17.68 69.88,17.37 68.81,17.37 68.43,17.75 52.05,17.75 51.44,18.36 44.27,18.36 43.51,17.6 40.39,17.6 v40.08,17.3 | v43.43,29.49 42.67,28.73 42.5,28.73 U1.P$75
  Bottom 0.152: X11.33 82.6,3.86 v82.6,6.63 82.6,14.02 v80.01,16.61 | v40.08,17.3 40.92,18.14 40.92,19.51 41.83,20.42 41.83,23.39 40.92,24.31 40.92,26.98 v43.43,29.49
PM4  (via drill 0.3)
  Top 0.152: X8.18 101.85,51.05 93.5,51.05 93.04,50.6 90.53,50.6 86.56,46.63 78.33,46.63 76.28,48.69 72.69,48.69 72.01,48.01 68.5,48.01 66.98,46.48 57.99,46.48 57.38,45.87 56.01,45.87 55.78,46.1 46.86,46.1 46.56,46.41 41.99,46.41 v41.68,46.1 | 14.63,21.41 v14.78,21.41 14.78,20.95 13.64,19.81 v13.18,19.81 | v14.63,25.07 23.47,25.07 23.7,24.84 23.77,24.77 23.93,24.61 28.96,24.61 29.18,24.84 29.87,25.53 32.38,25.53 32.69,25.83 36.12,25.83 36.65,26.36 39.55,26.36 41.25,28.06 U1.P$74 42.82,29.61 42.82,29.72 43.51,30.4 v43.59,30.4
  Bottom 0.152: v41.68,46.1 41.68,45.11 42.6,44.2 42.6,42.98 42.29,42.67 42.29,40.62 44.2,38.71 44.2,37.87 43.13,36.8 43.13,35.66 43.59,35.2 43.59,33.98 42.9,33.3 42.9,31.09 v43.59,30.4 | X11.92 10.36,2.74 10.36,5.11 11.96,6.71 11.96,15.16 12.88,16.08 12.88,17.83 13.18,18.14 v13.18,19.81 | v14.78,21.41 14.78,23.01 14.63,23.16 v14.63,25.07
PM5  (via drill 0.3)
  Top 0.152: X8.20 93.88,52.05 93.73,52.2 90.37,52.2 85.72,47.55 79.1,47.55 76.81,49.84 67.67,49.84 65.84,48.01 54.86,48.01 54.79,47.93 41.22,47.93 v41.07,48.01 | v13.18,25.76 15.16,25.76 15.54,25.38 23.7,25.38 23.93,25.15 24.16,24.92 28.8,24.92 29.18,25.3 29.03,25.15 29.72,25.83 32.23,25.83 32.54,26.14 35.97,26.14 36.5,26.67 39.32,26.67 39.47,26.82 U1.P$73 42.6,29.95 v42.6,30.4
  Bottom 0.152: X11.90 12.5,2.34 12.5,4.95 13.34,5.79 13.34,17.6 13.95,18.21 13.95,19.96 12.95,20.95 12.95,22.1 13.18,22.33 v13.18,25.76 | v42.6,30.4 42.6,33.45 43.28,34.14 43.28,34.9 42.82,35.36 42.82,37.03 43.81,38.02 43.81,38.56 41.99,40.46 41.99,42.82 42.29,43.2 42.29,43.97 41.07,45.19 v41.07,48.01
PM6  (via drill 0.3)
  Top 0.152: v15.01,26.52 15.85,25.68 24,25.68 24.46,25.22 28.65,25.22 29.57,26.14 32.08,26.14 32.38,26.44 35.81,26.44 36.65,27.28 v38.71,27.28 39.36,27.28 U1.P$72
  Bottom 0.152: v38.71,27.28 37.34,27.28 36.42,26.36 36.42,14.17 37.03,13.56 37.03,12.8 37.87,11.96 37.87,9.93 X7.20 | X11.88 13.89,1.27 12.8,2.36 12.8,4.72 13.64,5.56 13.64,17.37 15.54,19.28 15.54,25.98 v15.01,26.52
PM7  (via drill 0.3)
  Top 0.152: v16.15,26.36 16.69,26.36 17.07,25.98 24.23,25.98 24.69,25.53 28.5,25.53 28.73,25.76 29.41,26.44 31.93,26.44 32.23,26.75 35.66,26.75 36.8,27.89 39.4,27.89 U1.P$71 | v57.15,5.64 55.93,5.64 55.7,5.41 42.22,5.41 41.91,5.11 40.01,5.11 39.62,5.49 39.62,5.94 39.17,6.4 35.59,6.4 34.06,4.88 18.44,4.88 17.91,4.34 17.91,2.67 X11.86
  Bottom 0.152: v16.15,26.36 16.15,19.36 14.86,18.06 14.86,4.8 15.47,4.19 15.47,2.31 X11.86 | X7.4 v57.15,5.64
PN0  (via drill 0.3)
  Top 0.152: D2.A 25.68,6.24 | X11.85 18.26,5.56 24.99,5.56 25.67,6.24 25.68,6.24 | v25.91,20.88 26.59,20.88 30.18,17.3 36.8,17.3 38.02,18.52 42.82,18.52 43.59,19.28 45.41,19.28 46.33,20.19 47.85,20.19 48.77,21.11 48.77,22.48 50.29,24 50.29,25.6 50.67,25.98 51.17,25.98 U1.P$107 | 25.68,6.24 v25.68,6.25
  Bottom 0.152: v25.91,20.88 25.91,20.27 26.36,19.81 26.36,13.56 26.06,13.26 26.06,6.63 v25.68,6.25
PN1  (via drill 0.3)
  Top 0.152: D1.A v22.94,6.24 18.35,6.24 17.07,4.95 16.08,4.95 14.94,3.81 X11.87 | v25.07,21.64 26.29,21.64 30.33,17.6 36.5,17.6 37.72,18.82 42.6,18.82 43.36,19.58 45.26,19.58 46.1,20.5 47.7,20.5 48.46,21.26 48.46,22.63 49.99,24.16 49.99,25.76 50.52,26.29 51.43,26.29 U1.P$108
  Bottom 0.152: v25.07,21.64 25.07,19.36 25.91,18.52 25.91,14.78 22.86,11.73 22.86,9.83 23.09,9.6 23.09,8.08 22.86,7.85 22.86,6.31 v22.94,6.24
PN2  (via drill 0.3)
  Top 0.152: X9.16 105.36,8.89 104.32,7.85 99.9,7.85 99.14,8.61 92.43,8.61 91.36,7.54 86.56,7.54 85.95,8.15 77.04,8.15 76.81,7.92 v71.78,7.92 | v71.17,22.4 70.1,23.47 65.15,23.47 64.16,22.48 60.2,22.48 59.28,23.39 54.56,23.39 53.65,24.31 53.65,24.64 U1.P$109 | v12.72,14.86 12.72,16.84 16.61,20.73 23.39,20.73 27.43,16.69 40.39,16.69 41,17.3 43.74,17.3 44.5,18.06 51.21,18.06 51.82,17.45 68.28,17.45 68.66,17.07 v72.31,17.07
  Bottom 0.152: v71.17,22.4 71.78,21.79 71.78,17.07 | 71.78,17.07 v71.78,7.92 | X11.89 11.43,4.72 13.03,6.33 13.03,13.79 12.72,14.1 v12.72,14.86 | v72.31,17.07 71.78,17.07
PN3  (via drill 0.3)
  Top 0.152: X9.18 101.91,8.89 100.89,9.91 99.67,9.91 98.98,9.22 91.52,9.22 90.68,10.06 75.36,10.06 74.68,9.45 74.45,9.22 v73.15,9.22 | v72.24,22.4 71.55,23.01 70.71,23.77 64.85,23.77 63.86,22.78 60.35,22.78 59.44,23.7 54.79,23.7 54.01,24.48 54.01,24.84 U1.P$110 | v8.91,10.74 12.88,10.74 13.95,11.81 22.94,11.81 27.51,16.38 40.62,16.38 41.22,16.99 43.97,16.99 44.73,17.75 50.98,17.75 51.59,17.14 68.05,17.14 68.89,16.31 v72.85,16.31
  Bottom 0.152: v73.15,9.22 73.15,15.47 72.85,15.77 v72.85,16.31 72.85,16.76 73.15,17.07 73.15,20.27 72.24,21.18 v72.24,22.4 | X11.91 8.89,10.72 v8.91,10.74
PN4  (via drill 0.3)
  Top 0.152: v48.08,49.76 47.78,50.06 41,50.06 40.46,50.6 38.25,50.6 38.02,50.83 v38.02,50.98 | v52.27,26.36 52.73,26.67 53.11,26.29 53.12,26.29 U1.P$111 | v23.55,30.86 24.23,30.86 24.54,31.17 27.81,31.17 28.65,30.33 29.87,30.33 30.86,31.32 35.28,31.32 35.66,30.94 v36.2,30.94
  Bottom 0.152: v48.08,49.76 48.62,49.76 49.45,48.92 49.99,48.92 49.99,40.77 50.98,39.78 50.98,39.01 50.37,38.41 50.37,37.72 50.22,37.57 50.22,35.36 51.13,34.44 51.13,29.41 52.12,28.42 52.12,27.05 52.27,26.9 v52.27,26.36 | X6.19 38.02,53.42 v38.02,50.98 39.7,49.3 39.7,44.58 40.31,43.97 40.31,41.15 39.62,40.46 39.62,37.26 40.31,36.58 40.31,35.66 38.1,33.45 38.1,32.84 v36.2,30.94 | X11.81 21.57,4.27 21.57,6.02 20.12,7.47 20.12,10.97 19.58,11.51 18.75,11.51 17.14,13.11 17.14,18.06 20.73,21.64 20.73,22.86 23.55,25.68 v23.55,30.86
PN5  (via drill 0.3)
  Top 0.152: v49.3,49.99 48.84,50.44 41.22,50.44 40.84,50.83 40.84,53.14 X6.17 38.02,53.26 v35.66,53.26 | 52.77,27.28 v52.73,27.36 52.73,27.25 U1.P$112 | v19.89,31.32 20.27,31.7 22.33,31.7 23.93,33.3 26.75,33.3 27.28,33.83 27.28,34.44 28.5,35.66 30.1,35.66 v32,33.83
  Bottom 0.152: v49.3,49.99 49.99,49.3 50.14,49.3 50.29,49.15 50.29,40.92 51.28,39.93 51.28,38.86 50.67,38.25 50.67,35.36 51.44,34.59 51.44,29.57 52.73,28.27 v52.73,27.36 | X11.83 19.05,8.53 18.75,8.84 18.75,10.97 16.76,12.95 16.76,18.44 19.89,21.57 v19.89,31.32 | v32,33.83 32.08,33.83 32.69,34.37 32.69,37.8 35.51,40.69 35.51,49.61 35.05,50.06 35.05,52.65 v35.66,53.26
PP0  (via drill 0.3)
  Top 0.152: U1.P$118 56.32,27.05 v56.77,27.05
  Bottom 0.152: X6.5 53.57,53.57 53.57,44.12 54.1,43.59 54.1,32.92 55.63,31.39 55.63,30.63 56.46,29.79 56.46,27.36 v56.77,27.05 56.84,26.98 57.14,26.68 57.61,26.21 57.61,23.7 56.24,22.33 56.24,19.81 56.84,19.2 56.84,12.72 56.08,11.96 56.08,3.28 57.15,2.21 X11.54
PP1  (via drill 0.3)
  Top 0.152: v54.86,29.79 54.86,28.96 55.02,28.8 55.13,28.8 U1.P$119
  Bottom 0.152: X6.7 53.19,53.49 53.26,43.89 53.8,43.36 53.8,32.69 55.32,31.17 55.32,30.48 54.86,30.02 v54.86,29.79 55.7,29.79 55.93,29.57 55.93,27 57.3,25.7 57.3,23.85 55.93,22.48 55.93,19.66 56.54,19.05 56.54,12.95 55.78,12.19 55.78,3.28 54.61,2.11 X11.56
PP2  (via drill 0.3)
  Top 0.152: v77.65,24 77.65,23.55 75.89,21.79 70.87,21.79 69.49,23.16 65.46,23.16 64.47,22.1 58.6,22.1 57.91,22.78 52.1,22.78 U1.P$103 | X11.71 34.29,4.57 35.81,6.1 39.01,6.1 39.32,5.79 39.32,5.33 39.85,4.8 42.29,4.8 42.6,5.11 56.41,5.11 56.54,4.98 57.81,4.98 57.94,5.11 67.97,5.11 68.5,5.64 78.87,5.64 v79.17,5.94 | v77.8,9.45 78.33,8.91 100.33,8.91 X9.20
  Bottom 0.152: v77.65,24 77.65,21.41 76.05,19.81 76.05,17.14 77.65,15.54 77.65,9.6 v77.8,9.45 79.17,8.08 v79.17,5.94
PP3  (via drill 0.3)
  Top 0.152: X7.16 40.89,9.91 v32.77,9.91 | v59.13,22.71 58.52,22.71 58.14,23.09 52.36,23.09 U1.P$104 | v59.21,15.24 58.9,15.54 54.41,15.54 54.1,15.24 53.49,15.24 52.88,15.85 51.05,15.85 50.37,16.54 45.57,16.54 44.27,15.24 42.9,15.24 42.06,14.4 32.99,14.4 v32.38,13.79
  Bottom 0.152: X11.73 31.75,8.89 v32.77,9.91 32.38,10.29 v32.38,13.79 | v59.13,22.71 59.13,21.18 59.21,21.11 v59.21,15.24
PP4  (via drill 0.3)
  Top 0.152: 50.72,25.3 v50.9,25.38 50.9,24.92 51.05,24.77 51.25,24.77 U1.P$105 | v27.2,12.34 35.89,12.34 v36.42,12.8
  Bottom 0.152: v50.9,25.38 50.14,26.14 50.14,27.74 50.83,28.42 50.83,34.21 49.91,35.13 49.91,37.72 50.06,37.87 50.06,38.63 50.67,39.24 50.67,39.55 49.68,40.54 49.68,48.46 49.61,48.54 49.07,48.54 48.46,49.15 47.55,49.15 46.33,50.37 44.42,50.37 43.43,51.36 43.43,53.09 X6.15 40.46,53.16 40.46,45.26 41.91,43.81 41.91,43.36 40.69,42.14 40.69,41.07 39.93,40.31 39.93,37.41 40.69,36.65 40.69,35.36 38.48,33.15 38.48,32.46 37.03,31.01 37.03,30.33 36.65,30.02 36.65,27.13 36.12,26.59 36.12,13.95 36.42,13.64 v36.42,12.8 | X11.78 26.67,2.29 27.66,3.28 27.66,5.03 27.2,5.49 v27.2,12.34
PP5  (via drill 0.3)
  Top 0.152: v25.45,12.34 28.57,15.47 41.3,15.47 41.83,16 44.58,16 45.41,16.84 50.52,16.84 51.21,16.15 53.49,16.15 v53.8,15.85 | v53.42,23.7 52.89,23.7 U1.P$106
  Bottom 0.152: X11.80 24.13,2.11 25.15,3.12 25.15,5.18 24.77,5.56 24.77,7.32 25.45,8 v25.45,12.34 | X7.6 54.61,9.25 53.49,10.36 53.49,12.34 53.8,12.65 v53.8,15.85 53.8,16.31 54.63,17.14 54.63,22.25 53.42,23.39 v53.42,23.7
PQ0  (via drill 0.3)
  Top 0.152: X6.13 45.87,53.19 47.7,53.19 48.23,52.65 48.23,51.51 48.69,51.05 57.15,51.05 57.45,50.75 v57.91,50.75 | v59.89,34.29 58.52,34.29 58.22,34.59 57.99,34.59 U1.P$5
  Bottom 0.152: v57.91,50.75 60.2,48.46 60.2,43.43 59.59,42.82 59.59,35.43 59.89,35.13 v59.89,34.29 59.89,32.54 61.27,31.17 61.27,27.2 63.7,24.77 63.7,22.63 61.57,20.42 61.57,5.64 59.74,3.81 X11.51
PQ1  (via drill 0.3)
  Top 0.152: v58.67,34.98 57.8,34.98 U1.P$6 | 39.4,8.87 X7.18 40.31,7.95 40.31,7.47 40.77,7.01 43.43,7.01 43.66,7.24 45.41,7.24 45.72,6.93 48.23,6.93 49.07,6.1 53.8,6.1 54.33,6.63 58.6,6.63 v58.98,6.25
  Bottom 0.152: v58.67,34.98 58.67,32.99 58.83,32.84 58.83,31.47 58.98,31.32 58.98,30.25 59.05,30.18 59.05,23.62 59.97,22.71 59.97,17.53 60.58,16.92 60.58,12.12 60.73,11.96 60.73,8 v58.98,6.25 57.91,5.18 57.91,4.57 X11.53
PQ2  (via drill 0.3)
  Top 0.152: X7.12 46.99,8.87 | v53.11,7.62 52.73,7.62 52.65,7.54 51.36,7.54 50.98,7.92 50.14,7.92 50.06,7.85 49.15,7.85 48.77,8.23 47.65,8.23 X7.12 | v51.74,35.2 52.73,34.21 54.03,34.21 54.79,34.98 54.97,34.98 U1.P$11 | 47.02,8.91 X7.12 | R19.1 47.13,13.38 47.17,13.34 47.17,12.72 47.62,12.27 v48.23,12.27
  Bottom 0.152: v51.74,35.2 51.74,34.59 52.12,34.21 52.12,32.99 52.65,32.46 52.65,31.32 52.05,30.71 52.05,29.87 53.65,28.27 53.65,25.83 52.65,24.84 52.65,23.62 54.03,22.25 54.03,21.18 54.33,20.88 54.33,17.37 53.11,16.15 v53.11,7.62 54.71,7.62 55.4,6.93 55.4,4.57 X11.55 | v48.23,12.27 48.23,10.13 X7.12
PQ3  (via drill 0.3)
  Top 0.152: v50.6,7.32 49.23,7.32 48.69,7.85 46.48,7.85 45.49,8.84 44.96,8.84 X7.14 | v44.81,33.83 45.34,33.83 46.02,34.52 48.23,34.52 48.54,34.21 49.15,34.21 49.23,34.29 v49.68,34.29 | v49.84,39.32 50.29,39.32 51.07,40.09 U1.P$27 | v45.41,12.57 44.88,13.11 44.88,13.41 R20.1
